| IBIS file stm32l4r5_s5_ufbga132.ibs
[IBIS ver]   4.2
[File name]   stm32l4r5_s5_ufbga132.ibs
[File Rev]   1.0
[Date]   01-6-2017
[Source]   Data Created at STMicroelectronics
[Notes]   File originated from ELDO simulations.
[Disclaimer]   This information is for modeling purpose only and is
   not guaranted.
   The information is subject to change without notice.
[Copyright]   Copyright 2017 STMicroelectronics Inc.
|   Component stm32l4r5_s5_ufbga132
[Component] stm32l4r5_s5_ufbga132
[Manufacturer] STMicroelectronics
[Package]
| variable   typ   min   max
R_pkg   0.0   0.0   0.0
L_pkg   0.0H   0.0H   0.0H
C_pkg   0.0F   0.0F   0.0F
[Pin]  signal_name   model_name   R_pin   L_pin   C_pin
A1 PE3 io8prog2m25m50m120m_sudq_ft
A10 PA14 io8prog2m25m50m120m_sudq_ft
A11 PA13 io8prog2m25m50m120m_sudq_ft
A12 PA12 io8usblsfs_otg2
A2 PE1 io8prog2m25m50m120m_sudq_ft
A3 PB8 io8prog2m25m50m120m_sudq_i2c_ft
A4 PH3-BOOT0 io8prog2m25m50m120m_sudq_ft
A5 PD7 io8prog2m25m50m120m_sudq_ft
A6 PD5 io8prog2m25m50m120m_sudq_ft
A7 PB4 io8prog2m25m50m120m_sudq_i2c_ft
A8 PB3 io8prog2m25m50m120m_sudq_ft
A9 PA15 io8prog2m25m50m120m_sudq_ft
B1 PE4 io8prog2m25m50m120m_sudq_ft
B10 PC12 io8prog2m25m50m120m_sudq_ft
B11 PC10 io8prog2m25m50m120m_sudq_ft
B12 PA11 io8usblsfs_otg2
B2 PE2 io8prog2m25m50m120m_sudq_ft
B3 PB9 io8prog2m25m50m120m_sudq_i2c_ft
B4 PB7 io8prog2m25m50m120m_sudq_i2c_ft
B5 PB6 io8prog2m25m50m120m_sudq_i2c_ft
B6 PD6 io8prog2m25m50m120m_sudq_ft
B7 PD4 io8prog2m25m50m120m_sudq_ft
B8 PD3 io8prog2m25m50m120m_sudq_ft
B9 PD1 io8prog2m25m50m120m_sudq_ft
C1 PC13 io8prog2m25m50m120m_sudq_ft
C10 PC11 io8prog2m25m50m120m_sudq_ft
C11 VDDUSB power
C12 PA10 io8usb_id_otg20_lcd4_ft_ms
C2 PE5 io8prog2m25m50m120m_sudq_ft
C3 PE0 io8prog2m25m50m120m_sudq_ft
C4 VDD power
C5 PB5 io8prog2m25m50m120m_sudq_ft
C6 PG14 io8prog2m25m50m120m_sudq_i2c_ft
C7 PG13 io8prog2m25m50m120m_sudq_i2c_ft
C8 PD2 io8prog2m25m50m120m_sudq_ft
C9 PD0 io8prog2m25m50m120m_sudq_ft
D1 PC14-OSC32_IN io8prog2m25m50m120m_sudq_ft
D10 PA9 power
D11 PA8 io8prog2m25m50m120m_sudq_ft
D12 PC9 io8prog2m25m50m120m_sudq_ft
D2 PE6 io8prog2m25m50m120m_sudq_ft
D3 VSS gnd
D4 PF2 io8prog2m25m50m120m_sudq_ft
D5 PF1 io8prog2m25m50m120m_sudq_i2c_ft
D6 PF0 io8prog2m25m50m120m_sudq_i2c_ft
D7 PG12 io8prog2m25m50m120m_sudq_ft
D8 PG10 io8prog2m25m50m120m_sudq_ft
D9 PG9 io8prog2m25m50m120m_sudq_ft
E1 PC15-OSC32_OUT io8prog2m25m50m120m_sudq_ft
E10 PC8 io8prog2m25m50m120m_sudq_ft
E11 PC7 io8prog2m25m50m120m_sudq_ft
E12 PC6 io8prog2m25m50m120m_sudq_ft
E2 VBAT power
E3 VSS gnd
E4 PF3 io8prog2m25m50m120m_sudq_ft
E9 PG5 io8prog2m25m50m120m_sudq_ft
F1 PH0-OSC_IN io8prog2m25m50m120m_sudq_ft
F10 PG4 io8prog2m25m50m120m_sudq_ft
F11 VSS gnd
F12 VSS gnd
F2 VSS gnd
F3 PF4 io8prog2m25m50m120m_sudq_ft
F4 PF5 io8prog2m25m50m120m_sudq_ft
F6 VSS gnd
F7 VSS gnd
F9 PG3 io8prog2m25m50m120m_sudq_ft
G1 PH1-OSC_OUT io8prog2m25m50m120m_sudq_ft
G10 PG2 io8prog2m25m50m120m_sudq_ft
G11 VDD power
G2 VDD power
G3 PG11 io8prog2m25m50m120m_sudq_ft
G4 PG6 io8prog2m25m50m120m_sudq_ft
G6 VDD power
G7 VDDIO2 power
G9 PG1 io8prog2m25m50m120m_sudq_ft
H1 PC0 io8prog2m25m50m120m_sudq_i2c_ft
H10 PD15 io8prog2m25m50m120m_sudq_ft
H11 PD14 io8prog2m25m50m120m_sudq_ft
H12 PD13 io8prog2m25m50m120m_sudq_ft
H2 NRST ioreset_ft_v33
H3 VDD power
H4 PG7 io8prog2m25m50m120m_sudq_i2c_ft
H9 PG0 io8prog2m25m50m120m_sudq_ft
J1 VSSA/VREF- gnd
J10 PD12 io8prog2m25m50m120m_sudq_ft
J11 PD11 io8prog2m25m50m120m_sudq_ft
J12 PD10 io8prog2m25m50m120m_sudq_ft
J2 PC1 io8prog2m25m50m120m_sudq_i2c_ft
J3 PC2 io8prog2m25m50m120m_sudq_ft
J4 PA4 io8prog2m25m50m120m_sudq_ft
J5 PA7 io8prog2m25m50m120m_sudq_i2c_ft
J6 PG8 io8prog2m25m50m120m_sudq_i2c_ft
J7 PF12 io8prog2m25m50m120m_sudq_ft
J8 PF14 io8prog2m25m50m120m_sudq_i2c_ft
J9 PF15 io8prog2m25m50m120m_sudq_i2c_ft
K1 PG15 io8prog2m25m50m120m_sudq_ft
K10 PB15 io8prog2m25m50m120m_sudq_ft
K11 PB14 io8prog2m25m50m120m_sudq_i2c_ft
K12 PB13 io8prog2m25m50m120m_sudq_i2c_ft
K2 PC3 io8prog2m25m50m120m_sudq_ft
K3 PA2 io8prog2m25m50m120m_sudq_ft
K4 PA5 io8prog2m25m50m120m_sudq_ft
K5 PC4 io8prog2m25m50m120m_sudq_ft
K6 PF11 io8prog2m25m50m120m_sudq_ft
K7 PF13 io8prog2m25m50m120m_sudq_ft
K8 PD9 io8prog2m25m50m120m_sudq_ft
K9 PD8 io8prog2m25m50m120m_sudq_ft
L1 VREF+ power
L10 PB10 io8prog2m25m50m120m_sudq_i2c_ft
L11 PB11 io8prog2m25m50m120m_sudq_i2c_ft
L12 PB12 io8prog2m25m50m120m_sudq_ft
L2 PA0 io8prog2m25m50m120m_sudq_ft
L3 PA3 io8prog2m25m50m120m_sudq_ft
L4 PA6 io8prog2m25m50m120m_sudq_ft
L5 PC5 io8prog2m25m50m120m_sudq_ft
L6 PB2 io8prog2m25m50m120m_sudq_ft
L7 PE8 io8prog2m25m50m120m_sudq_ft
L8 PE10 io8prog2m25m50m120m_sudq_ft
L9 PE12 io8prog2m25m50m120m_sudq_ft
M1 VDDA power
M10 PE13 io8prog2m25m50m120m_sudq_ft
M11 PE14 io8prog2m25m50m120m_sudq_ft
M12 PE15 io8prog2m25m50m120m_sudq_ft
M2 PA1 io8prog2m25m50m120m_sudq_ft
|M3 OPAMP1_VINM nc
|M4 OPAMP2_VINM nc
M5 PB0 io8prog2m25m50m120m_sudq_ft
M6 PB1 io8prog2m25m50m120m_sudq_ft
M7 PE7 io8prog2m25m50m120m_sudq_ft
M8 PE9 io8prog2m25m50m120m_sudq_ft
M9 PE11 io8prog2m25m50m120m_sudq_ft
[Diff Pin]   inv_pin   vdiff   tdelay_typ  tdelay_min  tdelay_max
A12 B12 200mV   NA   NA   NA
[Model Selector] io8prog2m25m50m120m_sudq_ft
io8p00_sudq_ft_pd_lv  "SPEED00, PD=40kOhm - 1P8V"
io8p00_sudq_ft_pu_lv  "SPEED00, PU=40kOhm - 1P8V"
io8p00_sudq_ft_lv  "SPEED00 - 1P8V"
io8p00_sudq_ft_pd  "SPEED00, PD=40kOhm - 3P3V"
io8p00_sudq_ft_pu  "SPEED00, PU=40kOhm - 3P3V"
io8p00_sudq_ft  "SPEED00 - 3P3V"
io8p01_sudq_ft_pd_lv  "SPEED01, PD=40kOhm - 1P8V"
io8p01_sudq_ft_pu_lv  "SPEED01, PU=40kOhm - 1P8V"
io8p01_sudq_ft_lv  "SPEED01 - 1P8V"
io8p01_sudq_ft_pd  "SPEED01, PD=40kOhm - 3P3V"
io8p01_sudq_ft_pu  "SPEED01, PU=40kOhm - 3P3V"
io8p01_sudq_ft  "SPEED01 - 3P3V"
io8p10_sudq_ft_pd_lv  "SPEED10, PD=40kOhm - 1P8V"
io8p10_sudq_ft_pu_lv  "SPEED10, PU=40kOhm - 1P8V"
io8p10_sudq_ft_lv  "SPEED10 - 1P8V"
io8p10_sudq_ft_pd  "SPEED10, PD=40kOhm - 3P3V"
io8p10_sudq_ft_pu  "SPEED10, PU=40kOhm - 3P3V"
io8p10_sudq_ft  "SPEED10 - 3P3V"
io8p11_sudq_ft_pd_lv  "SPEED11, PD=40kOhm - 1P8V"
io8p11_sudq_ft_pu_lv  "SPEED11, PU=40kOhm - 1P8V"
io8p11_sudq_ft_lv  "SPEED11 - 1P8V"
io8p11_sudq_ft_pd  "SPEED11, PD=40kOhm - 3P3V"
io8p11_sudq_ft_pu  "SPEED11, PU=40kOhm - 3P3V"
io8p11_sudq_ft  "SPEED11 - 3P3V"
[Model Selector] io8prog2m25m50m120m_sudq_i2c_ft
io8prog_1v8_i2c_pd  "5V Tol GPIO 1.8V range i2c functionality with pull down"
io8prog_1v8_i2c_pu  "5V Tol GPIO 1.8V range i2c functionality with pull up"
io8prog_1v8_i2c  "5V Tol GPIO 1.8V range i2c functionality"
io8prog_3v3_i2c_pd  "5V Tol GPIO 3.3V range i2c functionality with pull down"
io8prog_3v3_i2c_pu  "5V Tol GPIO 3.3V range i2c functionality with pull up"
io8prog_3v3_i2c  "5V Tol GPIO 3.3V range i2c functionality"
io8prog_1v8_pd_00  "5V Tol GPIO 1.8V range with pd speed 00"
io8prog_1v8_pu_00  "5V Tol GPIO 1.8V range with pu speed 00"
io8prog_1v8_00  "5V Tol GPIO 1.8V range speed 00"
io8prog_3v3_pd_00  "5V Tol GPIO 3.3V range with pd speed 00"
io8prog_3v3_pu_00  "5V Tol GPIO 3.3V range with pu speed 00"
io8prog_3v3_00  "5V Tol GPIO 3.3V range speed 00"
io8prog_1v8_pd_01  "5V Tol GPIO 1.8V range with pd speed 01"
io8prog_1v8_pu_01  "5V Tol GPIO 1.8V range with pu speed 01"
io8prog_1v8_01  "5V Tol GPIO 1.8V range speed 01"
io8prog_3v3_pd_01  "5V Tol GPIO 3.3V range with pd speed 01"
io8prog_3v3_pu_01  "5V Tol GPIO 3.3V range with pu speed 01"
io8prog_3v3_01  "5V Tol GPIO 3.3V range speed 01"
io8prog_1v8_pd_10  "5V Tol GPIO 1.8V range with pd speed 10"
io8prog_1v8_pu_10  "5V Tol GPIO 1.8V range with pu speed 10"
io8prog_1v8_10  "5V Tol GPIO 1.8V range speed 10"
io8prog_3v3_pd_10  "5V Tol GPIO 3.3V range with pd speed 10"
io8prog_3v3_pu_10  "5V Tol GPIO 3.3V range with pu speed 10"
io8prog_3v3_10  "5V Tol GPIO 3.3V range speed 10"
io8prog_1v8_pd_11  "5V Tol GPIO 1.8V range with pd speed 11"
io8prog_1v8_pu_11  "5V Tol GPIO 1.8V range with pu speed 11"
io8prog_1v8_11  "5V Tol GPIO 1.8V range speed 11"
io8prog_3v3_pd_11  "5V Tol GPIO 3.3V range with pd speed 11"
io8prog_3v3_pu_11  "5V Tol GPIO 3.3V range with pu speed 11"
io8prog_3v3_11  "5V Tol GPIO 3.3V range speed 11"
[Model Selector] io8usb_id_otg20_lcd4_ft_ms
io8usbid_1v8_id_pu  "ID 1V8 range with pull up"
io8usbid_3v3_id_pu  "ID 3V3 range with pull up"
io8usbid_1v8_id  "ID 1V8 range"
io8usbid_3v3_id  "ID 3V3 range"
io8usbid_1v8_pd_00  "GPIO 1.8V range with pd speed 00"
io8usbid_1v8_pu_00  "GPIO 1.8V range with pu speed 00"
io8usbid_1v8_00  "GPIO 1.8V range speed 00"
io8usbid_3v3_pd_00  "GPIO 3.3V range with pd speed 00"
io8usbid_3v3_pu_00  "GPIO 3.3V range with pu speed 00"
io8usbid_3v3_00  "GPIO 3.3V range speed 00"
io8usbid_1v8_pd_01  "GPIO 1.8V range with pd speed 01"
io8usbid_1v8_pu_01  "GPIO 1.8V range with pu speed 01"
io8usbid_1v8_01  "GPIO 1.8V range speed 01"
io8usbid_3v3_pd_01  "GPIO 3.3V range with pd speed 01"
io8usbid_3v3_pu_01  "GPIO 3.3V range with pu speed 01"
io8usbid_3v3_01  "GPIO 3.3V range speed 01"
io8usbid_1v8_pd_10  "GPIO 1.8V range with pd speed 10"
io8usbid_1v8_pu_10  "GPIO 1.8V range with pu speed 10"
io8usbid_1v8_10  "GPIO 1.8V range speed 10"
io8usbid_3v3_pd_10  "GPIO 3.3V range with pd speed 10"
io8usbid_3v3_pu_10  "GPIO 3.3V range with pu speed 10"
io8usbid_3v3_10  "GPIO 3.3V range speed 10"
io8usbid_1v8_pd_11  "GPIO 1.8V range with pd speed 11"
io8usbid_1v8_pu_11  "GPIO 1.8V range with pu speed 11"
io8usbid_1v8_11  "GPIO 1.8V range speed 11"
io8usbid_3v3_pd_11  "GPIO 3.3V range with pd speed 11"
io8usbid_3v3_pu_11  "GPIO 3.3V range with pu speed 11"
io8usbid_3v3_11  "GPIO 3.3V range speed 11"
[Model Selector] io8usblsfs_otg2
usb_ls_pd  "USB Low Speed mode - Pull Down"
usb_ls_pu2  "USB Low Speed mode - Pull up 2"
usb_ls_pu  "USB Low Speed mode - Pull up"
usb_fs  "USB Low Speed mode"
usb_fs_pd  "USB Full Speed mode - Pull Down"
usb_fs_pu2  "USB Full Speed mode - Pull up 2"
usb_fs_pu  "USB Full Speed mode - Pull up"
[Model Selector] ioreset_ft_v33
ioreset_1v2_pu  "RESET 1.2V range with PU"
ioreset_1v2  "RESET 1.2V range"
ioreset_1v8_pu  "RESET 1.8V range with PU"
ioreset_1v8  "RESET 1.8V range"
ioreset_3v3_pu  "RESET 3.3V range with PU"
ioreset_3v3  "RESET 3.3V range"
| Models and submodels in the file (95): io8p00_sudq_ft_pd_lv (I/O), io8p00_sudq_ft_pu_lv (I/O), io8p00_sudq_ft_lv (I/O), io8p00_sudq_ft_pd (I/O), io8p00_sudq_ft_pu (I/O), io8p00_sudq_ft (I/O), io8p01_sudq_ft_pd_lv (I/O), io8p01_sudq_ft_pu_lv (I/O), io8p01_sudq_ft_lv (I/O), io8p01_sudq_ft_pd (I/O), io8p01_sudq_ft_pu (I/O), io8p01_sudq_ft (I/O), io8p10_sudq_ft_pd_lv (I/O), io8p10_sudq_ft_pu_lv (I/O), io8p10_sudq_ft_lv (I/O), io8p10_sudq_ft_pd (I/O), io8p10_sudq_ft_pu (I/O), io8p10_sudq_ft (I/O), io8p11_sudq_ft_pd_lv (I/O), io8p11_sudq_ft_pu_lv (I/O), io8p11_sudq_ft_lv (I/O), io8p11_sudq_ft_pd (I/O), io8p11_sudq_ft_pu (I/O), io8p11_sudq_ft (I/O), io8prog_1v8_i2c_pd (I/O), io8prog_1v8_i2c_pu (I/O), io8prog_1v8_i2c (I/O), io8prog_3v3_i2c_pd (I/O), io8prog_3v3_i2c_pu (I/O), io8prog_3v3_i2c (I/O), io8prog_1v8_pd_00 (I/O), io8prog_1v8_pu_00 (I/O), io8prog_1v8_00 (I/O), io8prog_3v3_pd_00 (I/O), io8prog_3v3_pu_00 (I/O), io8prog_3v3_00 (I/O), io8prog_1v8_pd_01 (I/O), io8prog_1v8_pu_01 (I/O), io8prog_1v8_01 (I/O), io8prog_3v3_pd_01 (I/O), io8prog_3v3_pu_01 (I/O), io8prog_3v3_01 (I/O), io8prog_1v8_pd_10 (I/O), io8prog_1v8_pu_10 (I/O), io8prog_1v8_10 (I/O), io8prog_3v3_pd_10 (I/O), io8prog_3v3_pu_10 (I/O), io8prog_3v3_10 (I/O), io8prog_1v8_pd_11 (I/O), io8prog_1v8_pu_11 (I/O), io8prog_1v8_11 (I/O), io8prog_3v3_pd_11 (I/O), io8prog_3v3_pu_11 (I/O), io8prog_3v3_11 (I/O), io8usbid_1v8_id_pu (Input), io8usbid_3v3_id_pu (Input), io8usbid_1v8_id (Input), io8usbid_3v3_id (Input), io8usbid_1v8_pd_00 (I/O), io8usbid_1v8_pu_00 (I/O), io8usbid_1v8_00 (I/O), io8usbid_3v3_pd_00 (I/O), io8usbid_3v3_pu_00 (I/O), io8usbid_3v3_00 (I/O), io8usbid_1v8_pd_01 (I/O), io8usbid_1v8_pu_01 (I/O), io8usbid_1v8_01 (I/O), io8usbid_3v3_pd_01 (I/O), io8usbid_3v3_pu_01 (I/O), io8usbid_3v3_01 (I/O), io8usbid_1v8_pd_10 (I/O), io8usbid_1v8_pu_10 (I/O), io8usbid_1v8_10 (I/O), io8usbid_3v3_pd_10 (I/O), io8usbid_3v3_pu_10 (I/O), io8usbid_3v3_10 (I/O), io8usbid_1v8_pd_11 (I/O), io8usbid_1v8_pu_11 (I/O), io8usbid_1v8_11 (I/O), io8usbid_3v3_pd_11 (I/O)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
